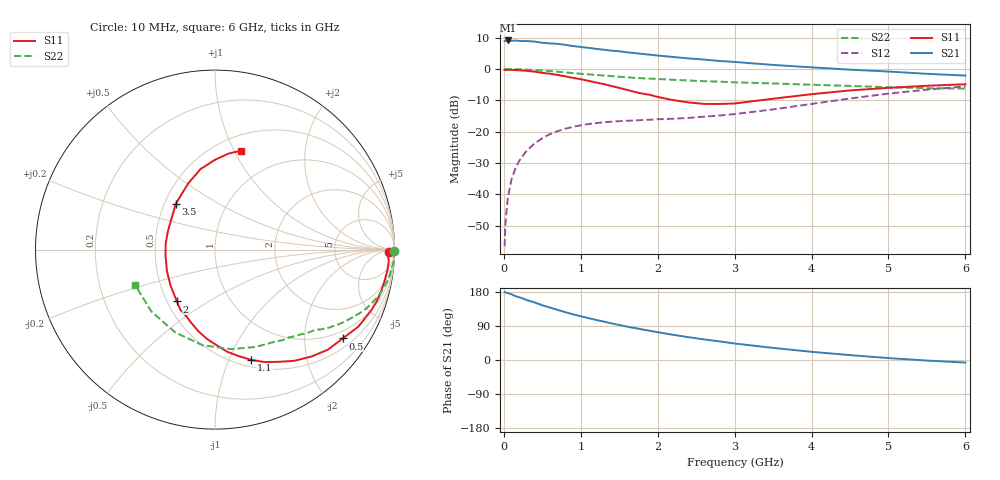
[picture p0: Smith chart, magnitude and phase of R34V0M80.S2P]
! SIEMENS Small Signal Semiconductors
! BFR181
! Si NPN RF Bipolar Junction Transistor in SOT23
! VCE = 4 V  IC = 0.8 mA
! Common Emitter S-Parameters:  May  1996
# GHz  S  MA  R  50
!  f  S11  S21  S12  S22
! GHz  MAG  ANG  MAG  ANG  MAG  ANG  MAG  ANG
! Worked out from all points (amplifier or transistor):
!   36 points, 10 MHz to 6 GHz, reference 50 ohm
!   highest |S21| = 9.1 dB at 50 MHz (marker M1)
!   |S21| within 3 dB of that: start of sweep to 1.316 GHz
!   unconditionally stable (mu >= 1): 2.139 GHz to 3.748 GHz
!   at 250 MHz: K = 0.13, MSG = 18.2 dB, |S12| = -27.5 dB
!   at 1.4 GHz: K = 0.70, MSG = 11.3 dB, |S12| = -16.8 dB
!   at 6 GHz: K = 0.89, MSG = 1.7 dB, |S12| = -5.6 dB
!   S11 on the Smith chart (normalised r, x): 10 MHz: 54, -25; 500 MHz: 0.76, -3.02; 1.1 GHz: 0.57, -1.21; 2 GHz: 0.56, -0.37; 3.5 GHz: 0.57, +0.33; 6 GHz: 0.65, +1.07
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0.01  0.9698 -0.8  2.787 179.6  0.0015 87.5  0.9999 -0.3
0.02  0.961 -1.3  2.804 178.5  0.0034 83.8  0.9984 -0.7
0.05  0.9705 -3.7  2.849 176.6  0.0085 88.3  0.9964 -1.7
0.1  0.9673 -7.1  2.807 173.3  0.0175 84.9  0.9996 -3.4
0.15  0.9602 -10.7  2.84 168.7  0.0259 82.2  0.9924 -5.2
0.2  0.9546 -14.0  2.804 165.5  0.0345 80.5  0.9878 -6.7
0.3  0.933 -21.5  2.79 158.0  0.0503 76.2  0.9778 -10.0
0.4  0.9065 -28.3  2.735 151.9  0.0651 71.2  0.9622 -13.1
0.5  0.867 -34.8  2.612 144.5  0.079 67.4  0.9448 -16.0
0.7  0.8025 -47.9  2.514 132.2  0.1024 59.7  0.9043 -21.3
0.8  0.7617 -54.4  2.425 126.1  0.1118 56.3  0.883 -23.5
1.1  0.6469 -71.8  2.175 110.5  0.1327 48.9  0.8215 -29.5
1.4  0.535 -88.7  1.958 96.6  0.1445 43.5  0.7698 -34.4
1.6  0.4648 -101.4  1.84 88.0  0.1498 41.7  0.7396 -36.9
2  0.3583 -126.3  1.637 73.3  0.1582 40.9  0.6936 -41.9
2.2  0.3195 -140.6  1.554 66.5  0.161 41.8  0.672 -44.7
2.6  0.2776 -173.1  1.414 54.4  0.1735 44.8  0.6385 -50.1
3  0.282 158.3  1.294 43.5  0.1912 48.0  0.6129 -56.7
3.5  0.3357 130.6  1.161 31.9  0.2269 50.7  0.588 -67.2
4.5  0.4554 100.3  0.975 12.9  0.3387 48.3  0.5368 -97.5
5.5  0.5402 82.0  0.838 -1.5  0.4686 35.9  0.4948 -135.8
6  0.571 75.1  0.785 -6.7  0.5268 27.8  0.4864 -156.0
